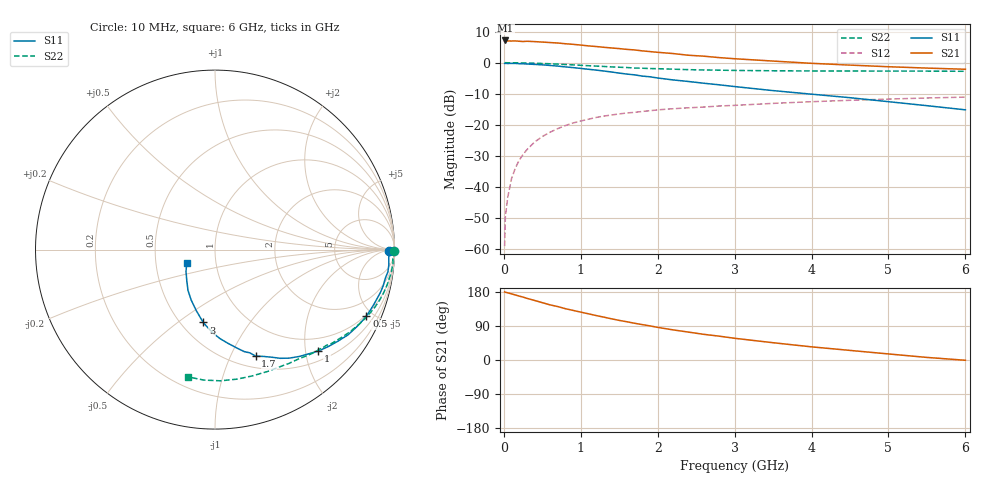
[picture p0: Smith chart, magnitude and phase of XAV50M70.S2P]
! SIEMENS Discrete & RF Semiconductors
! BFY180
! Si NPN RF Bipolar Junction Transistor in MICRO-X
! VCE = 0.5 V  IC = 0.7 mA
! Common Emitter S-Parameters:  May  1997
# GHz  S  MA  R  50
!  f  S11  S21  S12  S22
! GHz  MAG  ANG  MAG  ANG  MAG  ANG  MAG  ANG
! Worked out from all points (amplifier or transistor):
!   36 points, 10 MHz to 6 GHz, reference 50 ohm
!   highest |S21| = 7.2 dB at 20 MHz (marker M1)
!   |S21| within 3 dB of that: start of sweep to 1.667 GHz
!   unconditionally stable (mu >= 1): 2.828 GHz to end of sweep
!   at 250 MHz: K = 0.09, MSG = 18.2 dB, |S12| = -29.6 dB
!   at 1.4 GHz: K = 0.61, MSG = 10.8 dB, |S12| = -16.9 dB
!   at 6 GHz: K = 1.20, MAG = 1.8 dB, |S12| = -11.1 dB
!   S11 on the Smith chart (normalised r, x): 10 MHz: 64, -15; 500 MHz: 0.92, -4.57; 1 GHz: 0.70, -2.27; 1.7 GHz: 0.63, -1.25; 3 GHz: 0.64, -0.62; 6 GHz: 0.72, -0.11
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0.01  0.9707 -0.4  2.22 179.8  0.0011 91.5  0.9953 -0.3
0.02  0.973 -0.9  2.278 178.8  0.0033 93.0  0.997 -0.6
0.05  0.9689 -2.5  2.236 177.3  0.0067 88.5  0.9959 -1.4
0.1  0.9724 -5.0  2.231 174.5  0.0135 87.8  0.9922 -3.0
0.15  0.9713 -7.3  2.238 171.6  0.02 84.7  0.9945 -4.5
0.2  0.962 -9.7  2.211 168.6  0.0268 82.7  0.9918 -5.9
0.3  0.9521 -14.5  2.211 162.7  0.0395 79.4  0.9859 -8.8
0.5  0.9218 -23.8  2.147 151.3  0.0644 72.2  0.9696 -14.5
0.6  0.9012 -28.2  2.108 145.5  0.0755 69.1  0.9587 -17.2
0.8  0.8533 -36.8  2.017 135.4  0.0967 62.6  0.9329 -22.3
1  0.807 -44.4  1.92 126.3  0.1146 56.6  0.9058 -27.1
1.1  0.7813 -48.0  1.862 121.9  0.1225 54.2  0.8922 -29.2
1.4  0.7066 -59.0  1.724 108.7  0.1433 46.8  0.8538 -35.4
1.7  0.6352 -69.1  1.602 96.9  0.158 41.5  0.8188 -40.6
2  0.5656 -77.0  1.467 86.1  0.1733 36.9  0.7987 -45.5
2.2  0.5266 -82.2  1.401 79.5  0.1808 33.8  0.7843 -48.7
2.6  0.4654 -91.3  1.27 67.7  0.1924 29.2  0.7618 -54.3
3  0.4113 -99.2  1.156 57.3  0.2046 24.7  0.7486 -59.8
3.5  0.3541 -107.3  1.06 45.6  0.2204 20.6  0.7395 -66.6
4.5  0.2721 -123.6  0.913 25.3  0.2472 11.0  0.7321 -80.4
5.5  0.2024 -142.9  0.817 6.8  0.2693 1.7  0.7296 -94.9
6  0.1735 -155.0  0.782 -0.7  0.2782 -3.1  0.7252 -102.0
